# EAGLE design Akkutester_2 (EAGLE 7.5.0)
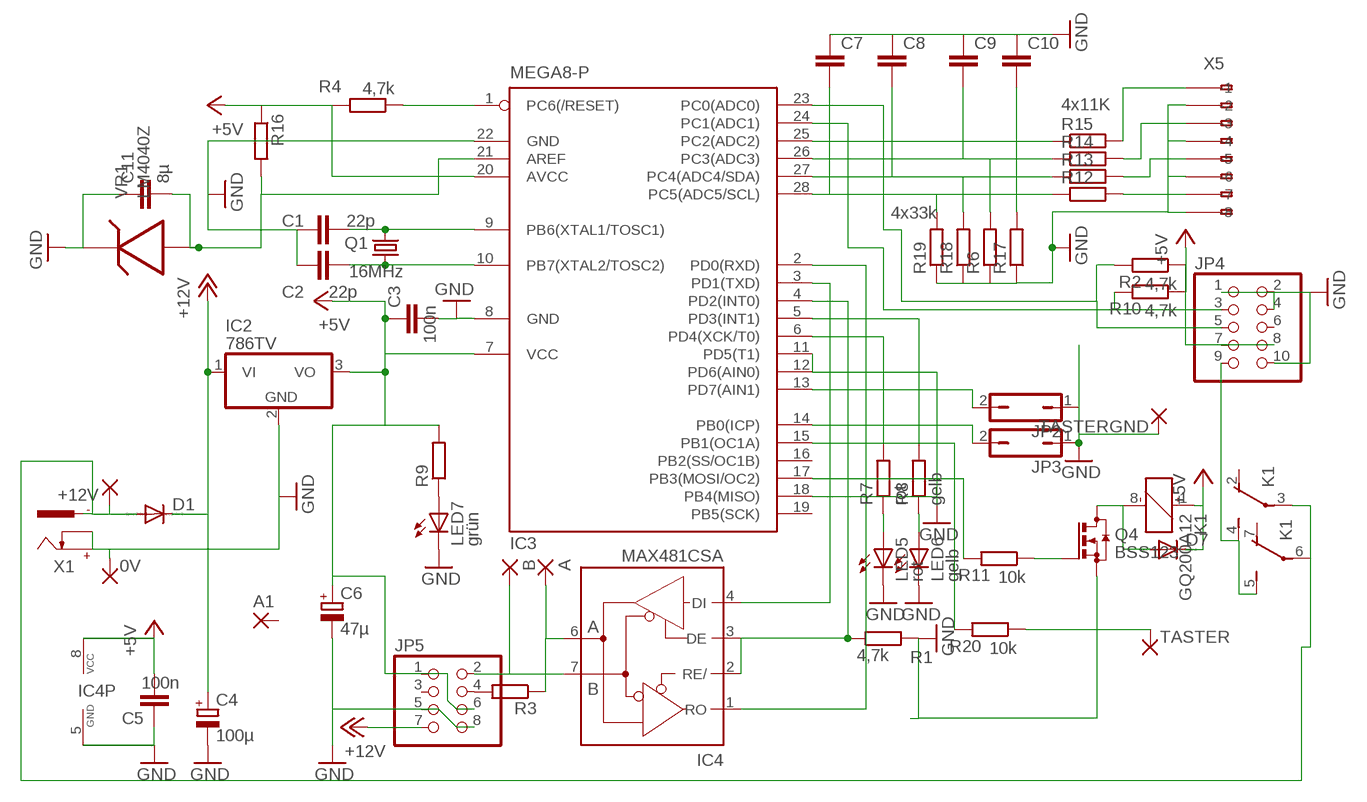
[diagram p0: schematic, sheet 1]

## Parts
0V  2,15/1,0  [2,15/1,0]
+12V  2,15/1,0  [2,15/1,0]
A  2,15/1,0  [2,15/1,0]
A1  2,15/1,0  [2,15/1,0]
B  2,15/1,0  [2,15/1,0]
C1  22p  C-EUC0603  [C0603]
C2  22p  C-EUC0603  [C0603]
C3  100n  C-EUC0603  [C0603]
C4  100µ  CPOL-EUSMCD  [SMC_D]
C5  100n  C-EU050-025X075  [C050-025X075]
C6  47µ  CPOL-EUSMCD  [SMC_D]
C7  C-EUC0603  [C0603]
C8  C-EUC0603  [C0603]
C9  C-EUC0603  [C0603]
C10  C-EUC0603  [C0603]
C11  8µ  C-EUC0603  [C0603]
D1  DIODE-DO214AA  [DO214AA]
D7  DIODE-SOD323-W  [SOD323-W]
IC2  786TV  [TO220V]
IC3  MEGA8-P  [DIL28-3]
IC4  MAX481CSA  [SO08]
JP2  JP1Q  [JP1]
JP3  JP1Q  [JP1]
JP4  PINHD-2X5  [2X05]
JP5  PINHD-2X4  [2X04]
K1  GQ200A12  [GN-A]
LED5  rot  LEDCHIPLED_0603  [CHIPLED_0603]
LED6  gelb  LEDCHIPLED_0603  [CHIPLED_0603]
LED7  grün  LEDCHIPLED_0603  [CHIPLED_0603]
Q1  16MHz  CRYSTALCTS406  [CTS406]
Q4  BSS123  [SOT23]
R1  4,7k  R-EU_R0603  [R0603]
R2  4,7k  R-EU_R0603  [R0603]
R3  R-EU_R1206  [R1206]
R4  4,7k  R-EU_R0603  [R0603]
R6  R-EU_R0603  [R0603]
R7  rot  R-EU_R0603  [R0603]
R8  gelb  R-EU_R0603  [R0603]
R9  R-EU_R0603  [R0603]
R10  4,7k  R-EU_R0603  [R0603]
R11  10k  R-EU_R0603  [R0603]
R12  R-EU_R0603  [R0603]
R13  R-EU_R0603  [R0603]
R14  R-EU_R0603  [R0603]
R15  4x11K  R-EU_R0603  [R0603]
R16  R-EU_R0603  [R0603]
R17  R-EU_R0603  [R0603]
R18  R-EU_R0603  [R0603]
R19  4x33k  R-EU_R0603  [R0603]
R20  10k  R-EU_R0603  [R0603]
TASTER  2,15/1,0  [2,15/1,0]
TASTERGND  2,15/1,0  [2,15/1,0]
VR1  LM4040Z  [TO92]
X1  737992-55  [737992-5]
X5  233-508  [233-508]

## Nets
+5V: C3.1 C5.2 C6.+ D7.C IC2.3(VO) IC3.7(VCC) IC3.20(AVCC) IC4.8(VCC) JP4.7 JP4.8 JP5.1 JP5.6 K1.1(1:+) R2.1 R4.2 R9.2 R10.1 R16.1
+12V: C4.+ D1.C IC2.1(VI) JP5.7
GND: 0V.1(P) C1.1 C2.1 C3.2 C4.- C5.1 C6.- C7.1 C8.1 C9.1 C10.1 C11.1 IC2.2(GND) IC3.8(GND) IC3.11(PD5(T1)) IC3.12(PD6(AIN0)) IC3.18(PB4(MISO)) IC3.22(GND) IC4.5(GND) JP2.1 JP3.1 JP4.1 JP4.2 JP4.4 JP4.10 JP5.5 JP5.8 LED5.C LED6.C LED7.C Q4.2(S) R1.2 R6.1 R17.1 R18.1 R19.1 TASTERGND.1(P) VR1.1 X1.+ X1.K X5.A2(-2) X5.A4(-4) X5.A6(-6) X5.A8(-8)
N$1: R20.1 TASTER.1(P)
N$2: IC3.2(PD0(RXD)) IC4.1(RO)
N$3: A.1(P) IC4.6(A) R3.1
N$4: B.1(P) IC4.7(B) JP5.2
N$5: C7.2 IC3.28(PC5(ADC5/SCL)) R12.1 R19.2
N$6: IC3.13(PD7(AIN1)) JP2.2
N$7: IC3.15(PB1(OC1A)) R20.2
N$8: LED7.A R9.1
N$9: C8.2 IC3.27(PC4(ADC4/SDA)) R13.1 R18.2
N$10: IC3.1(PC6(/RESET)) R4.1
N$11: C2.2 IC3.10(PB7(XTAL2/TOSC2)) Q1.1
N$12: C1.2 IC3.9(PB6(XTAL1/TOSC1)) Q1.3
N$13: IC3.3(PD1(TXD)) IC4.4(DI)
N$14: IC3.14(PB0(ICP)) JP3.2
N$15: IC3.4(PD2(INT0)) IC4.2(RE/) IC4.3(DE) R1.1
N$16: C9.2 IC3.26(PC3(ADC3)) R6.2 R14.1
N$17: C10.2 IC3.25(PC2(ADC2)) R15.1 R17.2
N$18: R15.2 X5.A1(-1)
N$19: R14.2 X5.A3(-3)
N$20: R13.2 X5.A5(-5)
N$21: R12.2 X5.A7(-7)
N$22: IC3.24(PC1(ADC1)) JP4.3 R10.2
N$23: JP5.4 R3.2
N$24: IC3.23(PC0(ADC0)) JP4.5 R2.2
N$25: D7.A K1.8(1:-) Q4.3(D)
N$27: C11.2 IC3.21(AREF) R16.2 VR1.2
N$28: Q4.1(G) R11.1
N$29: IC3.17(PB3(MOSI/OC2)) R11.2
N$31: +12V.1(P) D1.A K1.3(2:P) K1.6(3:P) X1.-1
N$32: JP4.9 K1.4(2:S) K1.5(3:S)
N$36: IC3.6(PD4(XCK/T0)) R7.2
N$37: IC3.5(PD3(INT1)) R8.2
N$38: LED5.A R7.1
N$39: LED6.A R8.1
Unconnected: A1.1(P) IC3.16(PB2(SS/OC1B)) IC3.19(PB5(SCK)) JP4.6 JP5.3 K1.2(2:O) K1.7(3:O) X1.-2 X5.B1(B-1) X5.B2(B-2) X5.B3(B-3) X5.B4(B-4) X5.B5(B-5) X5.B6(B-6) X5.B7(B-7) X5.B8(B-8)

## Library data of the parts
0V +12V A A1 B TASTER TASTERGND = wirepad:2,15/1,0: THROUGH-HOLE PAD
C1-C3 C5 C7-C11 = rcl:C-EU: CAPACITOR, European symbol
C4 C6 = rcl:CPOL-EU: POLARIZED CAPACITOR, European symbol
D1 D7 = diode:DIODE-: DIODE
IC2 = linear:78*: Positive VOLTAGE REGULATOR Source: http://cache.national.com/ds/LM/LM78L05.pdf http://www.fairchildsemi.com/ds/LM/LM7805.pdf
IC3 = atmel:MEGA8-P: MICROCONTROLLER 8 Kbytes FLASH, 1 kbytes SRAM, 512 bytes EEPROM, USART, 4-channel 10 bit ADC, 2-channel 8 bit ADC Pin compatible with Atmega48, ATMega88, ATMega168 Source: avr.lbr
IC4 = maxim:MAX481CSA: RS485 TRANSEIVER
JP2 JP3 = jumper:JP1Q: JUMPER
JP4 = pinhead:PINHD-2X5: PIN HEADER
JP5 = pinhead:PINHD-2X4: PIN HEADER
K1 = relay:GQ?*: ULTRA-SMALL PACKAGE FLAT POLARIZED RELAY NAiS Source: http://www.mew-europe.com/.. en_ds_61008_0000.pdf
LED5-LED7 = led:LED: LED
Q1 = crystal:CRYSTAL: CRYSTAL
Q4 = transistor-small-signal:BSS123: N-CHANNEL MOS FET
R1-R4 R6-R20 = rcl:R-EU_: RESISTOR, European symbol
VR1 = synthdiy:LM4040: Shunt VOLTAGE REG.
X1 = con-conrad:737992-55: FEMALE PRINT CONNECTOR DIN 45323 (34V/3A), ROKA, distributor Conrad
X5 = con-wago255:233-508: WAGO

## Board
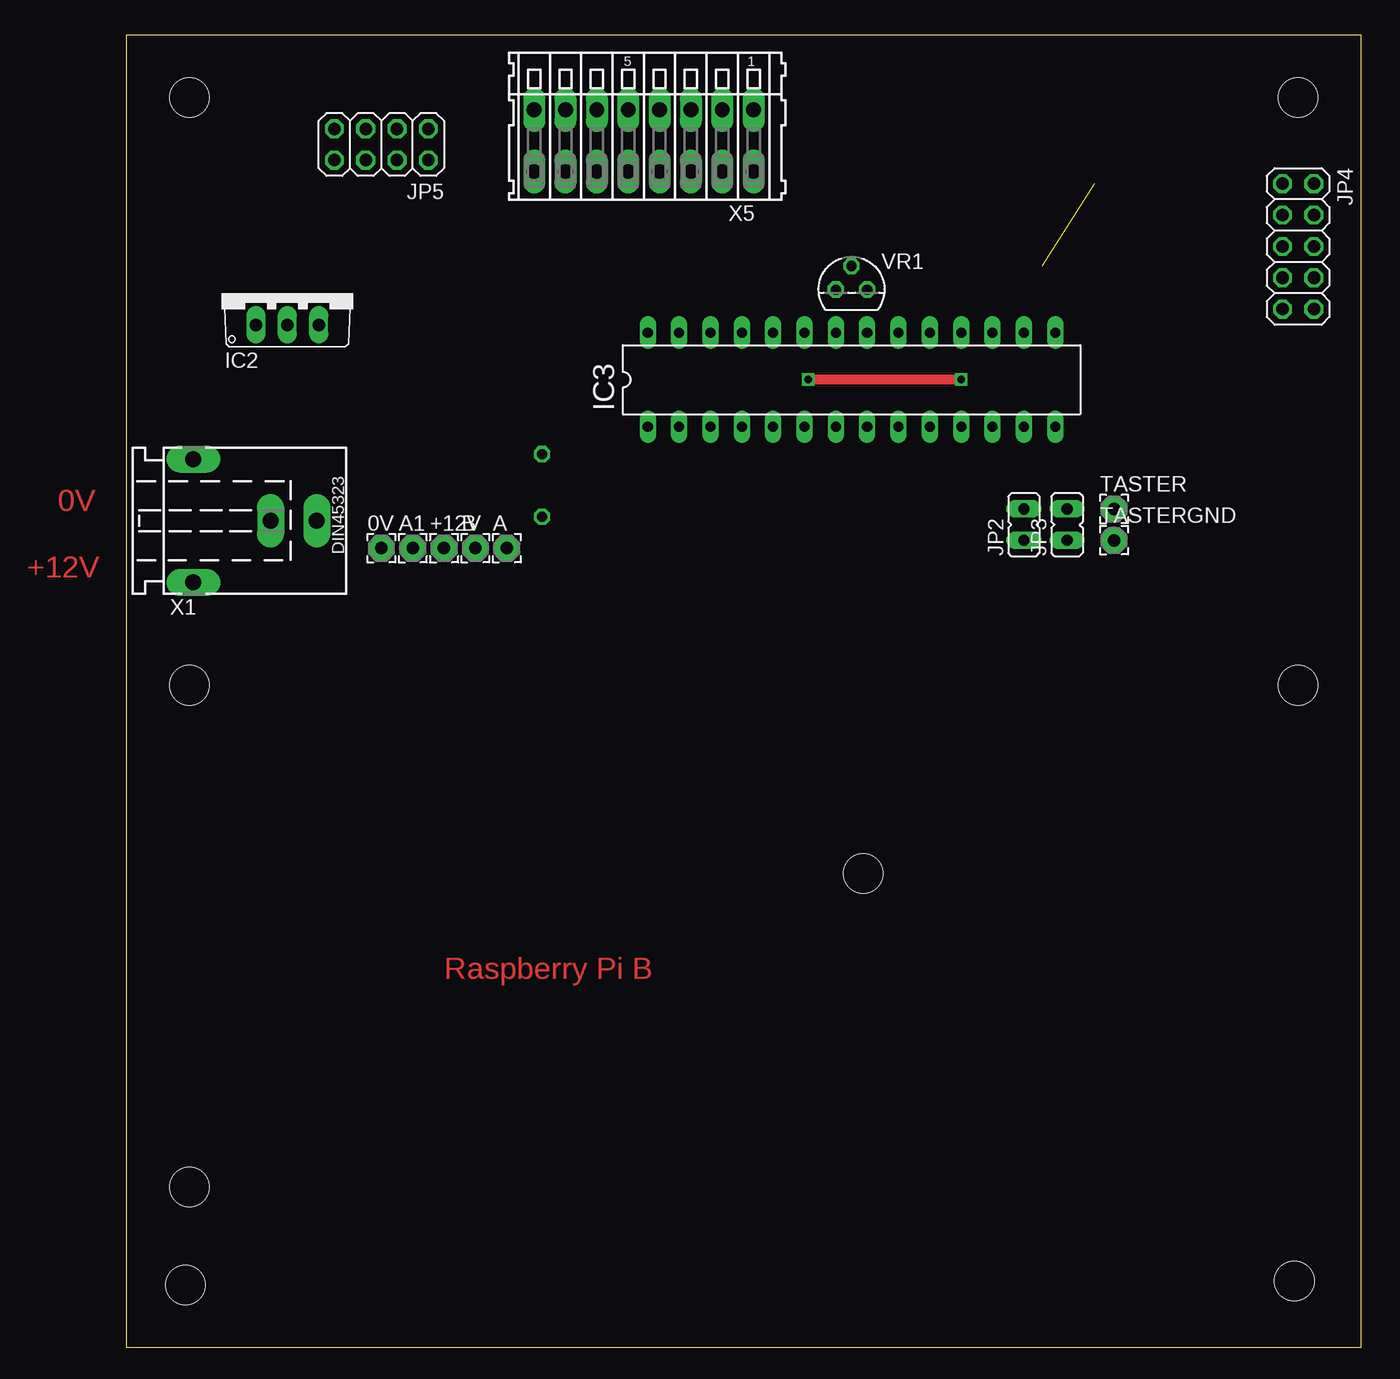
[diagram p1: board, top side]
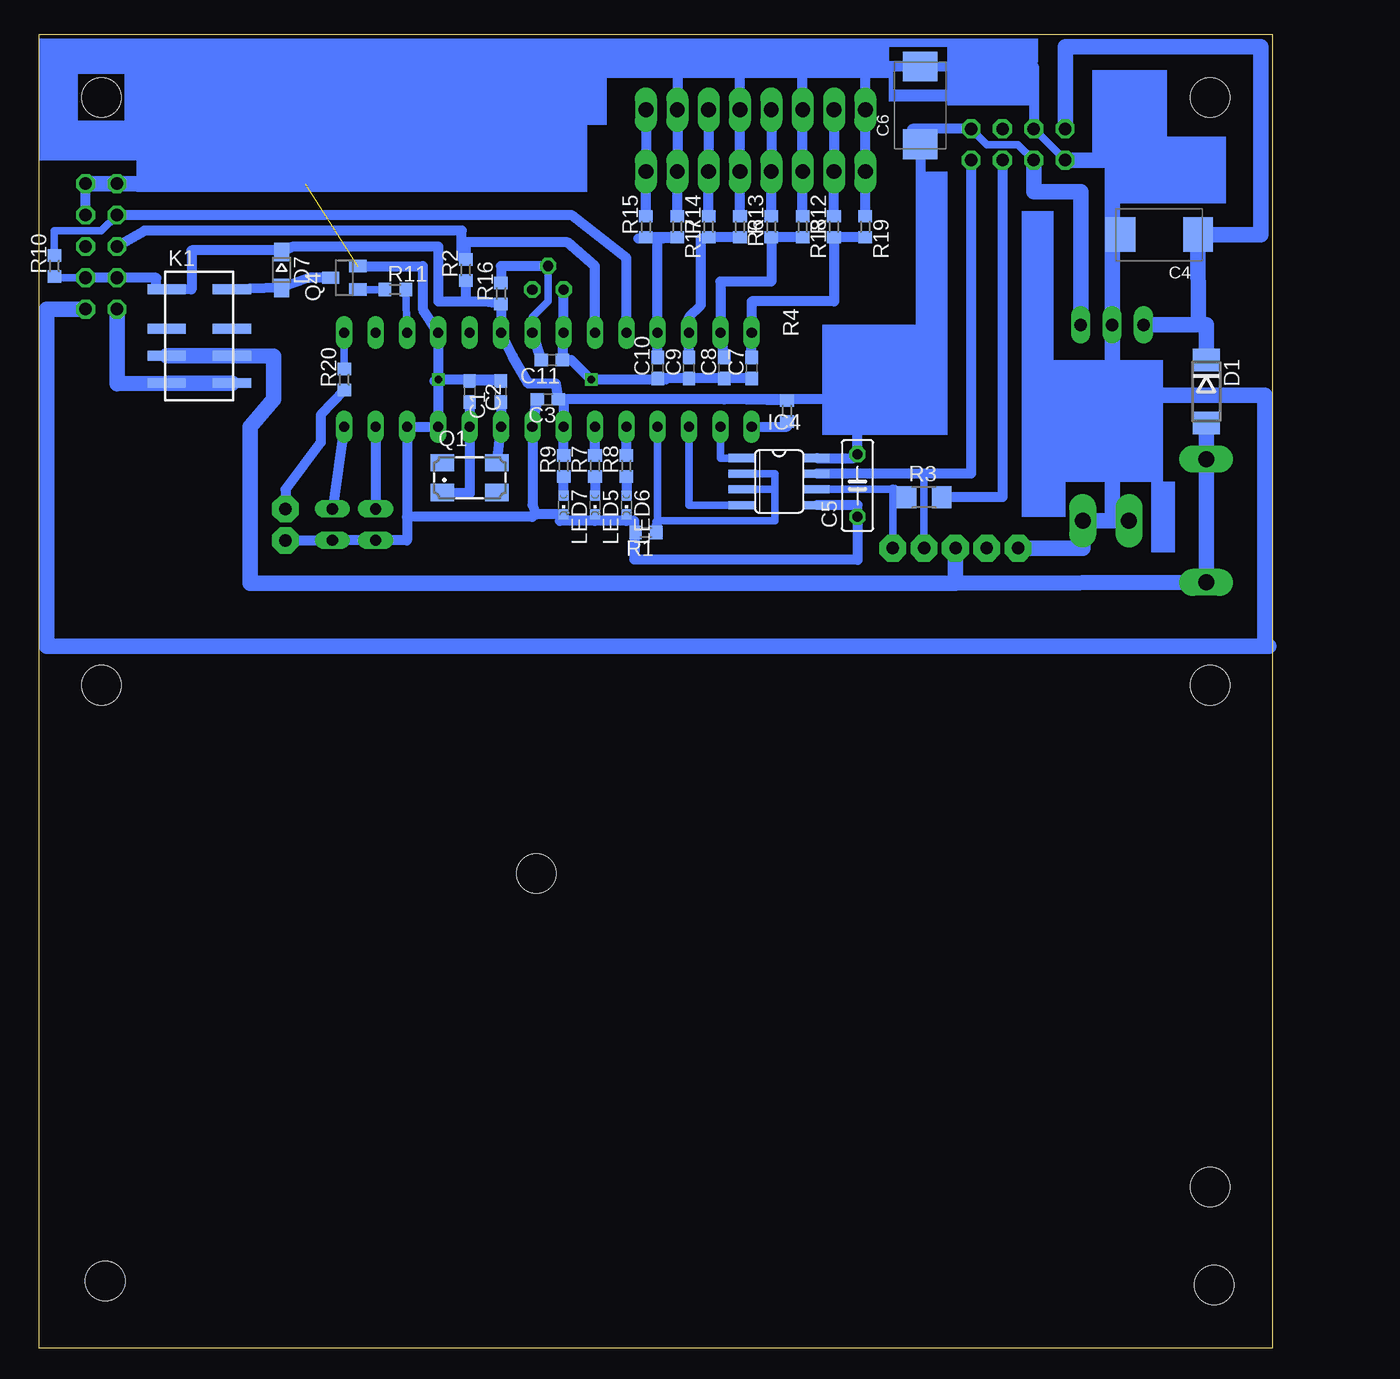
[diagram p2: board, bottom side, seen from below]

Size 100.01 x 106.36 mm. Coordinates in mm from the lower left corner, seen from the top.
Outline: 0,106.36 100.01,106.36 100.01,0 0,0 0,106.36
Copper layers (1*16): Top 0.035mm / dielectric 1.5mm / Bottom 0.035mm
Design rules "default": minimum track width 10mil, minimum drill 24mil, track to track 8mil, track to pad 8mil, pad to pad 8mil, via to via 8mil, smd to smd 8mil, copper to edge 40mil, drill to drill 8mil, minimum pad ring 10mil, minimum via ring 8mil, stop-mask expansion 4mil, vias tented up to drill 0mil, thermal gap 10mil
Holes 3.2 mm at 5.08,13.02 59.69,38.42 5.08,101.28 94.93,101.28 4.76,5.08 94.61,5.4 5.08,53.66 94.93,53.66

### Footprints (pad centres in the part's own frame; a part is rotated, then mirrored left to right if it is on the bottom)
2,15/1,0 = drill 1.016 pad 2.159 octagon: 1 0,0
C0603 = smd 1.1 x 1: 1 -0.85,0; 2 0.85,0
SMC_D = smd 2.4 x 2.8: + -3.15,0; - 3.15,0
C050-025X075 = drill 0.813 octagon: 1 -2.54,0; 2 2.54,0
DO214AA = smd 1.8 x 2.2: A 2.55,0; C -2.55,0
SOD323-W = smd 1.5 x 1.2: A 1.45,0; C -1.45,0
TO220V = drill 1.016 long: 1 -2.54,-2.54; 2 0,-2.54; 3 2.54,-2.54
DIL28-3 = drill 0.813 long: 1 -16.51,-3.81; 2 -13.97,-3.81; 3 -11.43,-3.81; 4 -8.89,-3.81; 5 -6.35,-3.81; 6 -3.81,-3.81; 7 -1.27,-3.81; 8 1.27,-3.81; 9 3.81,-3.81; 10 6.35,-3.81; 11 8.89,-3.81; 12 11.43,-3.81; 13 13.97,-3.81; 14 16.51,-3.81; 15 16.51,3.81; 16 13.97,3.81; 17 11.43,3.81; 18 8.89,3.81; 19 6.35,3.81; 20 3.81,3.81; 21 1.27,3.81; 22 -1.27,3.81; 23 -3.81,3.81; 24 -6.35,3.81; 25 -8.89,3.81; 26 -11.43,3.81; 27 -13.97,3.81; 28 -16.51,3.81
SO08 = smd 0.66 x 2.032: 1 -1.905,-3.073; 2 -0.635,-3.073; 3 0.635,-3.073; 4 1.905,-3.073; 5 1.905,3.073; 6 0.635,3.073; 7 -0.635,3.073; 8 -1.905,3.073
JP1 = drill 0.914 long: 1 0,-1.27; 2 0,1.27
2X05 = drill 1.016 octagon: 1 -5.08,-1.27; 2 -5.08,1.27; 3 -2.54,-1.27; 4 -2.54,1.27; 5 0,-1.27; 6 0,1.27; 7 2.54,-1.27; 8 2.54,1.27; 9 5.08,-1.27; 10 5.08,1.27
2X04 = drill 1.016 octagon: 1 -3.81,-1.27; 2 -3.81,1.27; 3 -1.27,-1.27; 4 -1.27,1.27; 5 1.27,-1.27; 6 1.27,1.27; 7 3.81,-1.27; 8 3.81,1.27
GN-A = smd 0.8 x 3.1: 1 -3.835,-2.65; 2 -0.635,-2.65; 3 1.565,-2.65; 4 3.765,-2.65; 5 3.765,2.65; 6 1.565,2.65; 7 -0.635,2.65; 8 -3.835,2.65
CHIPLED_0603 = smd 0.8 x 0.8: A 0,-0.75; C 0,0.75
CTS406 = smd 1.9 x 1.4: 1 -2.2,-1.2; 2 2.2,-1.2; 3 2.2,1.2; 4 -2.2,1.2
SOT23 = smd 1 x 1.4: 1 -0.95,-1.1; 2 0.95,-1.1; 3 0,1.1
R0603 = smd 1 x 1.1: 1 -0.85,0; 2 0.85,0
R1206 = smd 1.6 x 1.803: 1 -1.422,0; 2 1.422,0
TO92 = drill 0.813 octagon: 1 -1.27,0; 2 0,1.905; 3 1.27,0
737992-5 = drill 1.3 pad 2.184 long: + 0,10; -1 5,0; -2 -5,0; K 0,6.25
233-508 = drill 1.2 long: A1 -8.89,2.5; A2 -6.35,2.5; A3 -3.81,2.5; A4 -1.27,2.5; A5 1.27,2.5; A6 3.81,2.5; A7 6.35,2.5; A8 8.89,2.5; B1 -8.89,-2.5; B2 -6.35,-2.5; B3 -3.81,-2.5; B4 -1.27,-2.5; B5 1.27,-2.5; B6 3.81,-2.5; B7 6.35,-2.5; B8 8.89,-2.5

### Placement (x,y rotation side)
0V  20.64,64.77 0 top
+12V  25.72,64.77 0 top
A  30.8,64.77 0 top
A1  23.18,64.77 0 top
B  28.26,64.77 0 top
C1  62.55,77.47 270 bottom
C2  65.09,77.47 270 bottom
C3  58.74,76.83 180 bottom
C4  9.21,90.17 180 bottom
C5  33.66,69.85 90 bottom
C6  28.57,100.65 90 bottom
C7  42.23,79.38 90 bottom
C8  44.45,79.38 90 bottom
C9  47.31,79.38 90 bottom
C10  49.85,79.38 90 bottom
C11  58.42,80.01 180 bottom
D1  5.4,77.47 270 bottom
D7  80.33,87.31 270 bottom
IC2  13.02,85.41 0 top
IC3  58.74,78.42 0 top
IC4  40.01,70.17 270 bottom
JP2  72.71,66.67 0 top
JP3  76.2,66.67 0 top
JP4  94.93,89.22 270 top
JP5  20.64,97.47 180 top
K1  87,81.91 270 bottom
LED5  54.93,68.26 180 bottom
LED6  52.39,68.26 180 bottom
LED7  57.47,68.26 180 bottom
Q1  65.09,70.48 0 bottom
Q4  75.25,86.68 90 bottom
R1  50.8,66.04 180 bottom
R2  65.41,87.31 90 bottom
R3  28.26,68.9 0 bottom
R4  39.37,75.88 90 bottom
R6  43.18,90.81 270 bottom
R7  54.93,71.44 90 bottom
R8  52.39,71.44 90 bottom
R9  57.47,71.44 90 bottom
R10  98.74,87.63 90 bottom
R11  71.12,85.72 0 bottom
R12  35.56,90.81 90 bottom
R13  40.64,90.81 90 bottom
R14  45.72,90.81 90 bottom
R15  50.8,90.81 90 bottom
R16  62.55,85.41 90 bottom
R17  48.26,90.81 270 bottom
R18  38.1,90.81 270 bottom
R19  33.02,90.81 270 bottom
R20  75.25,78.42 90 bottom
TASTER  80.01,67.94 0 top
TASTERGND  80.01,65.41 0 top
VR1  58.74,85.72 0 top
X1  5.4,66.99 270 top
X5  41.91,97.79 180 top

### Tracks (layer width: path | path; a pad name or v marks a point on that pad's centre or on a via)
+5V
  Bottom 0.61: JP5.6 20.64,97.47 23.18,97.47 JP5.1 | R10.1 98.42,86.68 JP4.8
  Bottom 0.813: R4.2 44.45,76.83 | 44.45,76.83 57.47,76.83 | 57.47,76.83 IC3.7 R9.2 | 33.97,72.39 C5.2 | C5.2 33.66,76.83 | 33.66,76.83 44.45,76.83 | JP5.1 29.21,98.74 C6.+ 28.57,76.83 33.66,76.83 | 57.47,76.83 C3.1 58.1,78.1 60.33,78.1 61.59,80.33 IC3.20 R16.1 63.82,84.77 65.41,84.77 | R2.1 65.41,84.77 | 65.41,84.77 67.63,84.77 67.63,89.22 79.38,89.22 D7.C 80.01,88.9 87.63,88.9 87.63,85.72 K1.1 90.49,85.72 90.49,86.68 JP4.7 JP4.8 | IC4.8 33.97,72.07 C5.2
  Bottom 1.27: IC2.3 15.56,93.66 19.37,93.66 JP5.6
+12V
  Bottom 1.27: 6.03,82.87 5.4,82.87 D1.C | IC2.1 6.03,82.87 | 6.03,82.87 C4.+ 0.95,90.17 0.95,105.41 16.83,105.41 JP5.7
GND  (via drill 0.6)  (1 unrouted)
  Top 0.813: v67.63,78.42 v55.24,78.42
  Bottom 0.61: JP5.8 JP5.5
  Bottom 0.813: IC4.5 33.66,68.26 C5.1 33.66,63.82 51.73,63.84 R1.2 51.75,66.99 52.39,66.99 | 59.69,67.51 LED7.C 57.78,66.99 54.93,66.99 | 59.69,67.51 60.01,67.31 70.17,67.31 | 70.17,67.31 IC3.12 IC3.11 v67.63,78.42 | C2.1 C1.1 62.55,78.42 v67.63,78.42 | v67.63,78.42 IC3.18 68.9,84.14 68.9,87.63 Q4.2 | VR1.1 IC3.22 C11.1 56.83,80.01 v55.24,78.42 49.21,78.42 C10.1 C9.1 C8.1 C7.1 | IC3.8 C3.2 59.69,76.83 IC3.8 | 70.17,67.31 70.17,65.4 JP2.1 JP3.1 TASTERGND.1 | R19.1 X5.A8 33.02,103.82 | 35.56,103.82 38.1,103.82 | 38.1,103.82 43.18,103.82 | 43.18,103.82 48.26,103.82 | 48.26,103.82 X5.A2 R17.1 | 43.18,103.82 X5.A4 R6.1 | R18.1 X5.A6 38.1,103.82 | 48.26,103.82 78.42,103.82 78.42,95.57 | 35.56,103.82 33.02,103.82 | 33.02,103.82 19.37,103.82 JP5.5 | C6.- 35.56,103.82 | 52.39,66.99 54.93,66.99 | LED5.C 54.93,66.99 | LED6.C 52.39,66.99 | IC3.8 60.01,68.26 59.69,67.51 | 67.94,78.32 v67.63,78.42 | JP4.4 JP4.2
  Bottom 1.27: 12.38,66.99 X1.K 13.02,66.99 | 13.02,66.99 X1.+ 15.4,64.77 0V.1 | 13.02,90.17 IC2.2 13.02,77.15 | C4.- 13.02,90.17 | 13.02,77.15 13.02,66.99 | JP5.8 13.02,96.2 13.02,90.17 | JP4.2 JP4.1 78.42,94.3 78.42,95.57 | JP4.10 99.38,84.14 99.38,56.83 0.64,56.83 | 0.32,56.83 0.64,56.83 | 0.64,56.83 0.64,77.15 13.02,77.15
N$1
  Bottom 0.813: R20.1 77.15,75.56 77.15,73.34 80.01,69.53 TASTER.1
N$2
  Bottom 0.61: IC4.1 44.77,72.07 IC3.2
N$3
  Bottom 0.61: A.1 30.8,69.53 IC4.6
  Bottom 0.813: R3.1 30.8,69.53
N$4
  Bottom 0.61: B.1 28.26,70.8
  Bottom 0.813: JP5.2 24.45,70.8 28.26,70.8 IC4.7
N$5
  Bottom 0.813: R19.2 R12.1 35.56,84.77 42.23,84.77 IC3.28 C7.2
N$6
  Bottom 0.813: IC3.13 JP2.2
N$7
  Bottom 0.61: R20.2 IC3.15
N$8
  Bottom 0.813: LED7.A R9.1
N$9
  Bottom 0.813: R18.2 R13.1 40.64,86.36 44.77,86.36 IC3.27 C8.2
N$10
  Bottom 0.813: IC3.1 39.37,74.61 R4.1
N$11
  Bottom 0.813: C2.2 IC3.10 65.09,69.22 66.02,69.22 Q1.1
N$12
  Bottom 0.813: C1.2 IC3.9 62.57,74.61 Q1.3
N$13
  Bottom 0.61: IC3.3 47.31,68.26 IC4.4
N$14
  Bottom 0.813: IC3.14 JP3.2
N$15
  Bottom 0.61: 40.32,69.53 IC4.3 | IC4.2 40.32,70.8 40.32,69.53 | 40.32,69.53 40.32,66.99 49.85,66.99 IC3.4
  Bottom 0.813: R1.1 49.85,66.99
N$16
  Bottom 0.813: R6.2 R14.1 46.35,89.85 46.35,84.46 47.31,83.5 IC3.26 C9.2
N$17
  Bottom 0.813: C10.2 IC3.25 49.85,89.85 R17.2 R15.1 51.44,89.85
N$18
  Bottom 0.813: R15.2 X5.A1 50.8,100.96
N$19
  Bottom 0.813: R14.2 X5.A3 45.72,100.96
N$20
  Bottom 0.813: R13.2 X5.A5 40.64,100.96
N$21
  Bottom 0.813: R12.2 X5.A7 35.56,100.65
N$22
  Bottom 0.61: JP4.3 94.93,90.49 98.74,90.49 R10.2
  Bottom 0.813: IC3.24 52.39,88.27 56.83,91.76 JP4.3
N$23
  Bottom 0.813: JP5.4 21.91,68.9 R3.2
N$24
  Bottom 0.813: IC3.23 54.93,87.63 57.15,89.53 65.41,89.53 R2.2 65.72,88.27 65.72,90.49 91.44,90.49 JP4.5
N$25
  Bottom 0.813: Q4.3 78.11,86.68 D7.A K1.8
N$27
  Bottom 0.61: IC3.21 60.01,83.5 58.74,84.77 VR1.2
  Bottom 0.813: VR1.2 62.55,87.63 R16.2 | C11.2 IC3.21
N$28
  Bottom 0.61: R11.1 73.98,85.72 Q4.1
N$29
  Bottom 0.61: IC3.17 R11.2
N$31
  Bottom 1.27: D1.A X1.-1 25.72,61.91 | K1.3 K1.6 80.96,80.33 80.96,76.83 82.87,74.61 82.87,61.91 25.72,61.91 | +12V.1 25.72,61.91
N$32
  Bottom 1.27: K1.5 K1.4 93.66,78.1 JP4.9
N$36
  Bottom 0.813: R7.2 IC3.6
N$37
  Bottom 0.813: R8.2 IC3.5
N$38
  Bottom 0.813: R7.1 LED5.A
N$39
  Bottom 0.813: R8.1 LED6.A
(copper drawn outside any net)
  shapes: Bottom area x23

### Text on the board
Top: 0V | +12V | Raspberry Pi B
